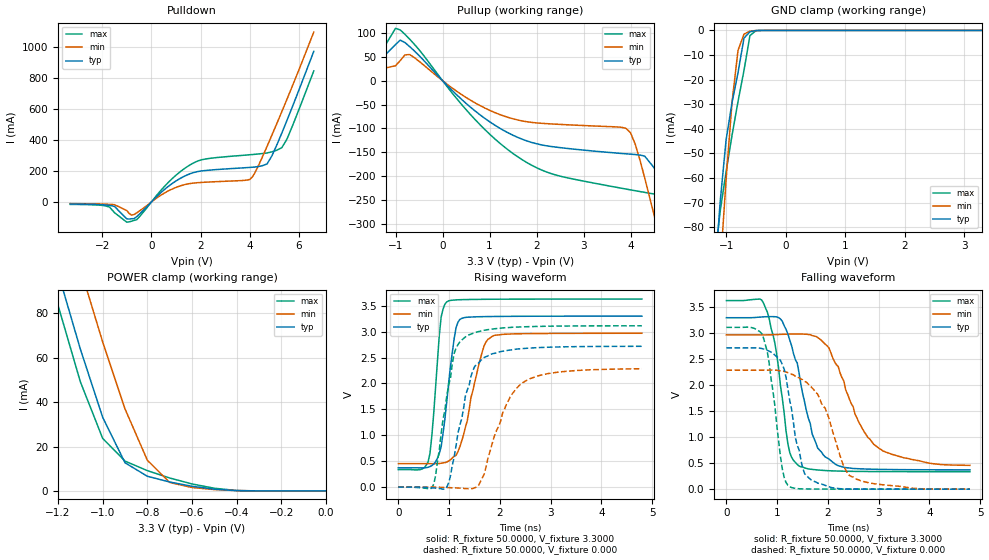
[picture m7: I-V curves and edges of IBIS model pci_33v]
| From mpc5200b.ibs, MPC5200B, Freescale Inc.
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|   Model pci_33v
[Model]   pci_33v
Model_type   I/O
Polarity   Non-Inverting
Enable   Active-High
Vinl =   0.8000V
Vinh =   2.0000V
Vmeas =   1.5000V
C_comp   2.1096pF   1.4802pF   2.7108pF
[Temperature Range]   27.0000   0.1250k   -40.0000
[Voltage Range]   3.3000V   2.9700V   3.6300V
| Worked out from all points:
|   slope of the pulldown table from 0 to 0.495 V, typ, clamps not added: 6.52 ohm
|   slope of the pullup table from 0 to 0.495 V, typ, clamps not added: 10.5 ohm
|   GND clamp passes 1 mA (typ) near -0.62 V on its own axis
|   POWER clamp passes 1 mA (typ) near -0.52 V on its own axis
|   rising waveform, R_fixture 50.0000, V_fixture 3.3000: 20-80 % time 210ps typ, 345ps min, 151ps max; typ from 0.372 V to 3.3 V
|   rising waveform, R_fixture 50.0000, V_fixture 0.000: 20-80 % time 352ps typ, 523ps min, 292ps max; typ from 0 V to 2.72 V
|   falling waveform, R_fixture 50.0000, V_fixture 3.3000: 20-80 % time 438ps typ, 706ps min, 276ps max; typ from 3.3 V to 0.372 V
|   falling waveform, R_fixture 50.0000, V_fixture 0.000: 20-80 % time 303ps typ, 509ps min, 235ps max; typ from 2.72 V to 0 V
[Pulldown]
| voltage   I(typ)   I(min)   I(max)
-3.3V     -12.76mA   -10.52mA   -15.49mA
-1.9V     -18.87mA   -13.92mA   -23.7mA
-1.5V     -28.97mA   -17.44mA   -69.11mA
-1V       -109.5mA   -55.4mA    -130.7mA
-800mV    -108.2mA   -84.83mA   -124.2mA
600mV     89.86mA    64.06mA    112.2mA
1.6V      184.2mA    120.1mA    242.5mA
4V        223.5mA    146.3mA    305.4mA
4.7V      246mA      359.3mA    317.1mA
5.3V      445.4mA    584.1mA    351.1mA
5.7V      603.7mA    738.3mA    478.9mA
6.6V      974.1mA    1.099A     847.7mA
[Pullup]
| voltage   I(typ)   I(min)   I(max)
-3.3V     13.78mA    14.26mA    16.13mA
-1.5V     25.86mA    20.34mA    28.53mA
-900mV    84.78mA    41.91mA    106.1mA
700mV     -63.96mA   -46.93mA   -82.16mA
1.8V      -126.3mA   -86.05mA   -171.7mA
3.9V      -153mA     -99.6mA    -226.7mA
4.1V      -154.6mA   -133.1mA   -230.2mA
4.5V      -182.1mA   -280.7mA   -237.1mA
4.7V      -217.3mA   -360.9mA   -241.2mA
4.9V      -285.2mA   -442.6mA   -265.7mA
5.1V      -363.7mA   -525.3mA   -294.7mA
6.6V      -995.6mA   -1.157A    -848.3mA
[GND_clamp]
| voltage   I(typ)   I(min)   I(max)
-3.3V     -981.7mA   -1.007A    -969.3mA
-1.2V     -103.3mA   -135mA     -94.78mA
-1.1V     -69.66mA   -96.96mA   -73.57mA
-1V       -44.44mA   -60.49mA   -57.28mA
-900mV    -29.26mA   -28.95mA   -42.5mA
-800mV    -17.16mA   -8.11mA    -28.87mA
-700mV    -3.155mA   -1.52mA    -16.29mA
-600mV    -543.7uA   -295.5uA   -2.097mA
-500mV    -57.86uA   -49uA      -141uA
-400mV    -4.573uA   -7.081uA   -5.584uA
3.3V      1.734nA    36.38uA    1.392nA
[POWER_clamp]
| voltage   I(typ)   I(min)   I(max)
-3.3V     947.4mA    944.7mA    949.5mA
-1.3V     134.5mA    170.5mA    121.3mA
-1.2V     98.3mA     134.9mA    83.61mA
-1.1V     63.86mA    100.2mA    49.15mA
-1V       33.15mA    67.07mA    23.65mA
-900mV    12.68mA    36.94mA    13.44mA
-800mV    6.604mA    13.81mA    9.138mA
-700mV    4.019mA    3.816mA    5.825mA
-600mV    2.098mA    1.54mA     3.147mA
-500mV    780.7uA    610.9uA    1.207mA
-400mV    131uA      150.3uA    180.7uA
0V        1.734nA    10.2nA     5.073nA
[Ramp]
| variable   typ   min   max
dV/dt_r   1.6274/0.3585n   1.3530/0.5016n   1.8667/0.3046n
dV/dt_f   1.7552/0.4386n   1.4305/0.6160n   1.9758/0.2802n
R_load = 50.0000
[Rising Waveform]
R_fixture = 50.0000
V_fixture = 3.3000
V_fixture_min = 2.9700
V_fixture_max = 3.6300
| time   V(typ)   V(min)   V(max)
0s        371.8mV    451.8mV    336.1mV
587.8ps   382.4mV    451.8mV    487.6mV
661.2ps   415.3mV    451.4mV    993.6mV
844.9ps   780.3mV    459.9mV    3.287V
955.1ps   1.649V     483.3mV    3.575V
1.102ns   2.873V     594.7mV    3.611V
1.176ns   3.183V     683.8mV    3.616V
1.653ns   3.29V      2.603V     3.625V
1.837ns   3.293V     2.901V     3.626V
4.8ns     3.3V       2.97V      3.63V
[Rising Waveform]
R_fixture = 50.0000
V_fixture = 0.000
| time   V(typ)   V(min)   V(max)
0s        18.94nV    50.68nV    45.24nV
698ps     -17.96mV   -937.4uV   53.9mV
955.1ps   -1.153mV   -9.266mV   1.758V
1.102ns   586mV      -15.65mV   2.585V
1.359ns   1.875V     -31.81mV   2.927V
1.506ns   2.33V      -14.41mV   2.978V
1.69ns    2.501V     242.1mV    3.027V
2.057ns   2.623V     1.433V     3.072V
2.461ns   2.675V     2.022V     3.093V
4.8ns     2.718V     2.284V     3.114V
[Falling Waveform]
R_fixture = 50.0000
V_fixture = 3.3000
V_fixture_min = 2.9700
V_fixture_max = 3.6300
| time   V(typ)   V(min)   V(max)
0s        3.3V       2.97V      3.63V
734.7ps   3.317V     2.97V      3.574V
955.1ps   3.319V     2.974V     2.811V
1.249ns   2.868V     2.985V     704.7mV
1.433ns   2.233V     2.986V     443.6mV
1.8ns     791.3mV    2.918V     369.3mV
2.167ns   469.3mV    2.394V     349.7mV
2.608ns   393.1mV    1.292V     341.5mV
3.012ns   380.9mV    782.6mV    338.7mV
4.8ns     372.1mV    458.4mV    336.2mV
[Falling Waveform]
R_fixture = 50.0000
V_fixture = 0.000
| time   V(typ)   V(min)   V(max)
0s        2.719V     2.29V      3.114V
698ps     2.707V     2.29V      2.993V
844.9ps   2.656V     2.291V     2.409V
1.102ns   2.401V     2.271V     391.6mV
1.249ns   1.705V     2.223V     44.54mV
1.506ns   399mV      2.105V     4.761mV
1.69ns    164.3mV    1.948V     3.044mV
1.947ns   72.86mV    1.557V     1.64mV
2.425ns   2.093mV    263.1mV    654.4uV
4.8ns     16.19uV    229.4uV    7.595uV
